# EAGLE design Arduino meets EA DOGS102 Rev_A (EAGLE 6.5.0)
Assembly variants: 3.3V monochrome, 3.3V RGB
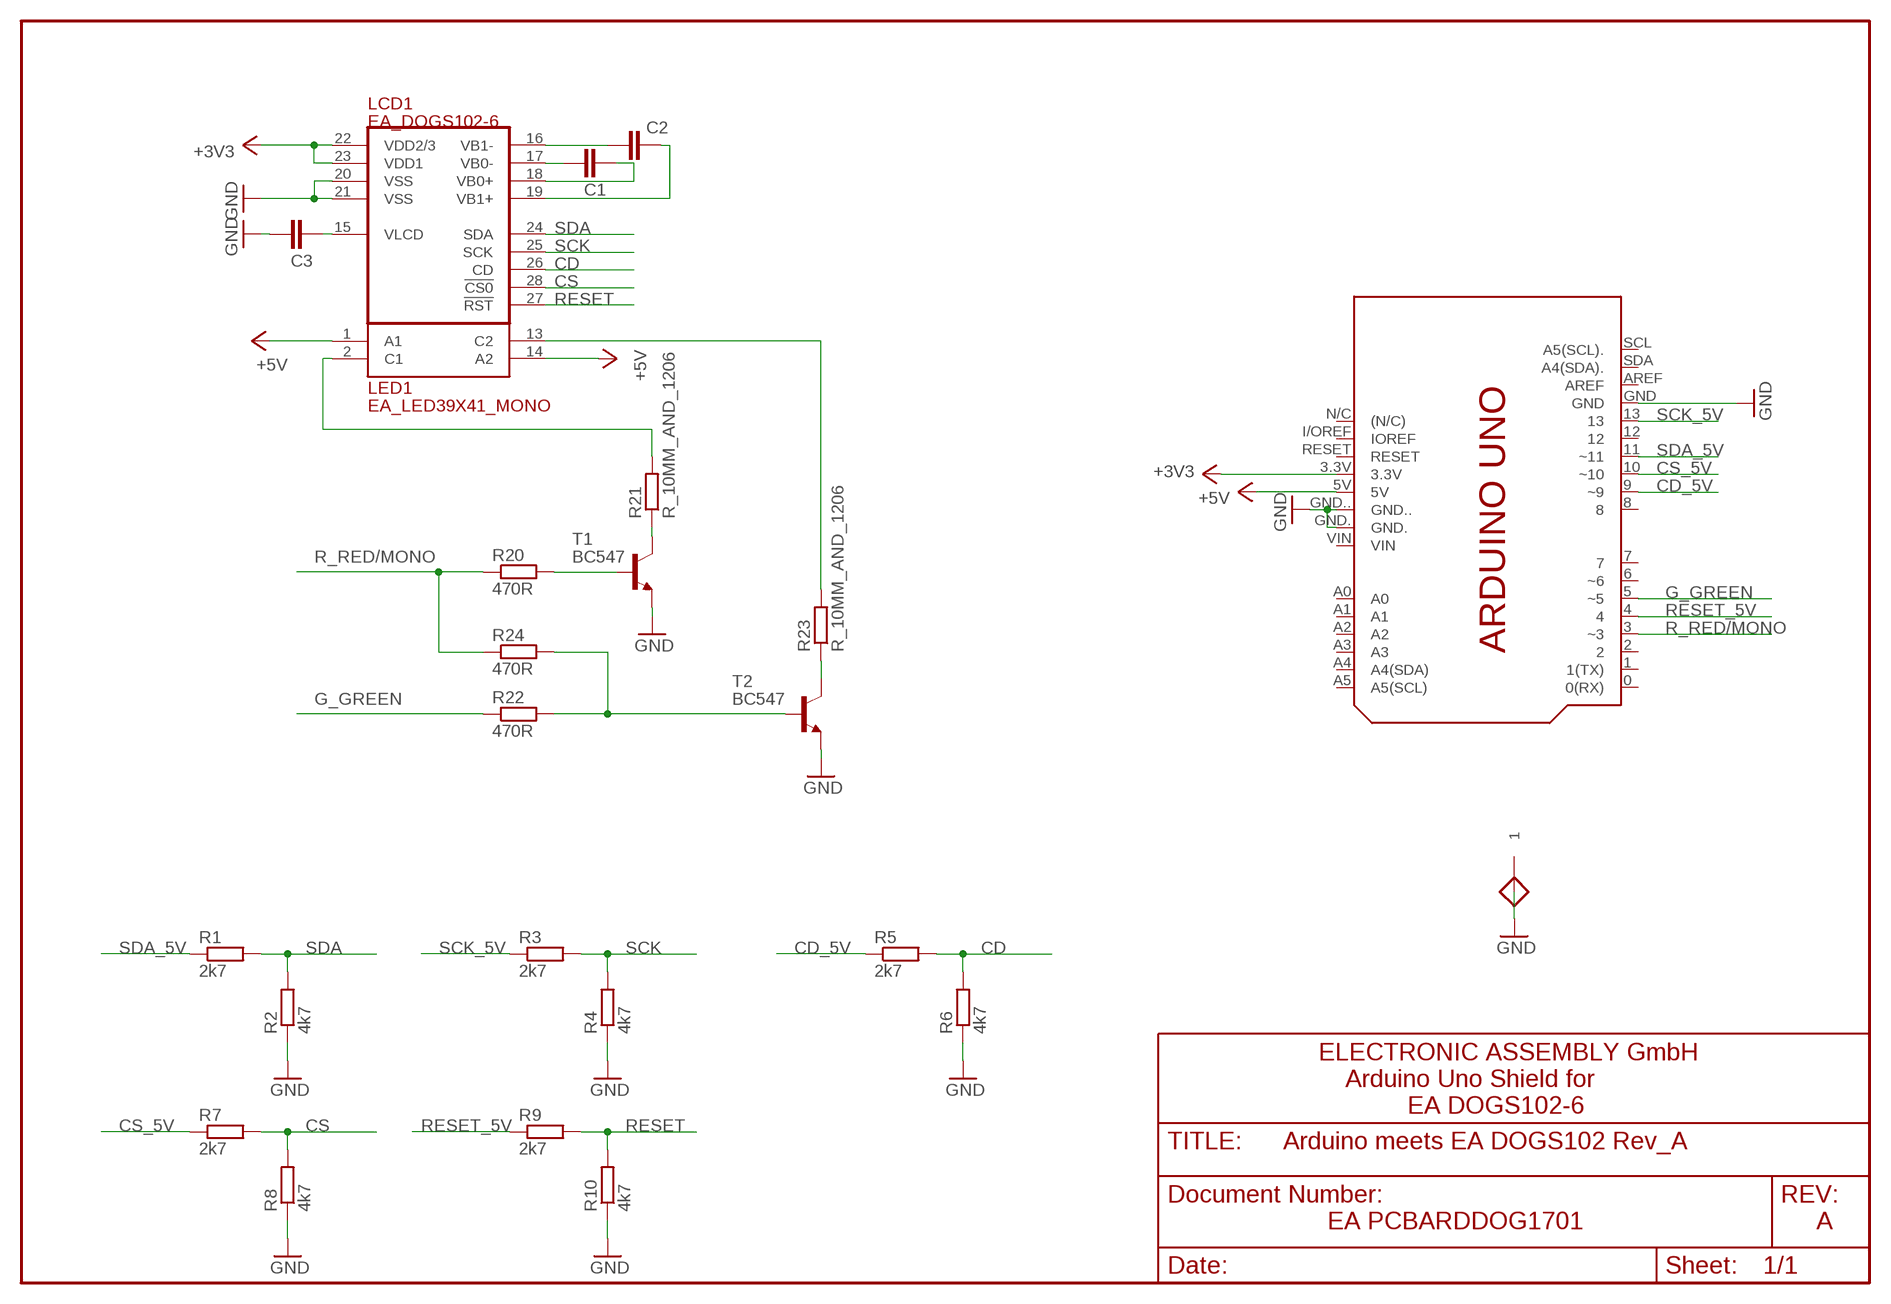
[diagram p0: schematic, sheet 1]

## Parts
C1  1uF  C_5MM_AND_1206  [C_5MM_AND_1206]
C2  1uF  C_5MM_AND_1206  [C_5MM_AND_1206]
C3  1uF  C_5MM_AND_1206  [C_5MM_AND_1206]
GND  PAD55/35  [PAD55/35]
LCD1  EA_DOGS102-6  [EA_DOGS102-6]
LED1  EA_LED39X41_MONO  [EA_LED39X41]
PCB1  ARDUINO_UNO_SHIELD  [ARDUINO_UNO_SHIELD]
R1  2k7  R_10MM_AND_1206  [R_10MM_AND_1206]
R2  4k7  R_10MM_AND_1206  [R_10MM_AND_1206]
R3  2k7  R_10MM_AND_1206  [R_10MM_AND_1206]
R4  4k7  R_10MM_AND_1206  [R_10MM_AND_1206]
R5  2k7  R_10MM_AND_1206  [R_10MM_AND_1206]
R6  4k7  R_10MM_AND_1206  [R_10MM_AND_1206]
R7  2k7  R_10MM_AND_1206  [R_10MM_AND_1206]
R8  4k7  R_10MM_AND_1206  [R_10MM_AND_1206]
R9  2k7  R_10MM_AND_1206  [R_10MM_AND_1206]
R10  4k7  R_10MM_AND_1206  [R_10MM_AND_1206]
R20  470R  R_10MM_AND_1206  [R_10MM_AND_1206]
R21  R_10MM_AND_1206  [R_10MM_AND_1206]
R22  470R  R_10MM_AND_1206  [R_10MM_AND_1206]  (not fitted in variant 3.3V monochrome)
R23  R_10MM_AND_1206  [R_10MM_AND_1206]
R24  470R  R_10MM_AND_1206  [R_10MM_AND_1206]  (not fitted in variant 3.3V RGB)
T1  BC547  [TO92]
T2  BC547  [TO92]

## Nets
+3V3: LCD1.22(VDD2/3) LCD1.23(VDD1) PCB1.3.3V
+5V: LED1.1(A1) LED1.14(A2) PCB1.5V
CD: LCD1.26(CD) R5.2 R6.2
CD_5V: PCB1.9(~9) R5.1
CS: LCD1.28(!CS0!) R7.2 R8.2
CS_5V: PCB1.10(~10) R7.1
G_GREEN: PCB1.5(~5) R22.1
GND: C3.2 GND.1 LCD1.20(VSS) LCD1.21(VSS) PCB1.GND PCB1.GND. PCB1.GND.. R2.1 R4.1 R6.1 R8.1 R10.1 T1.1(E) T2.1(E)
N$1: C1.2 LCD1.17(VB0-)
N$2: C2.2 LCD1.16(VB1-)
N$3: C1.1 LCD1.18(VB0+)
N$4: C2.1 LCD1.19(VB1+)
N$5: C3.1 LCD1.15(VLCD)
N$6: R21.1 T1.3(C)
N$7: LED1.2(C1) R21.2
N$12: R20.2 T1.2(B)
N$14: LED1.13(C2) R23.2
N$16: R23.1 T2.3(C)
N$17: R22.2 R24.2 T2.2(B)
R_RED/MONO: PCB1.3(~3) R20.1 R24.1
RESET: LCD1.27(!RST!) R9.2 R10.2
RESET_5V: PCB1.4 R9.1
SCK: LCD1.25(SCK) R3.2 R4.2
SCK_5V: PCB1.13 R3.1
SDA: LCD1.24(SDA) R1.2 R2.2
SDA_5V: PCB1.11(~11) R1.1
Unconnected: PCB1.0(0(RX)) PCB1.1(1(TX)) PCB1.2 PCB1.6(~6) PCB1.7 PCB1.8 PCB1.12 PCB1.A0 PCB1.A1 PCB1.A2 PCB1.A3 PCB1.A4(A4(SDA)) PCB1.A5(A5(SCL)) PCB1.AREF PCB1.I/OREF(IOREF) PCB1.N/C((N/C)) PCB1.RESET PCB1.SCL(A5(SCL).) PCB1.SDA(A4(SDA).) PCB1.VIN

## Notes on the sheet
- ELECTRONIC ASSEMBLY GmbH
- Arduino Uno Shield for
- EA DOGS102-6
- EA PCBARDDOG1701 | A

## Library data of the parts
C1-C3 = EA:C_5MM_AND_1206
GND = EA:PAD55/35
LCD1 = EA:EA_DOGS102-6
LED1 = EA:EA_LED39X41_MONO: Manufacturer: ELECTRONIC ASSEMBLY GmbH EA LED39x41-A EA LED39x41-W EA LED39x41-GR
PCB1 = E14_Arduino:ARDUINO_UNO_SHIELD
R1-R10 R20-R24 = EA:R_10MM_AND_1206
T1 T2 = transistor-npn:BC547: NPN TRANSISTOR

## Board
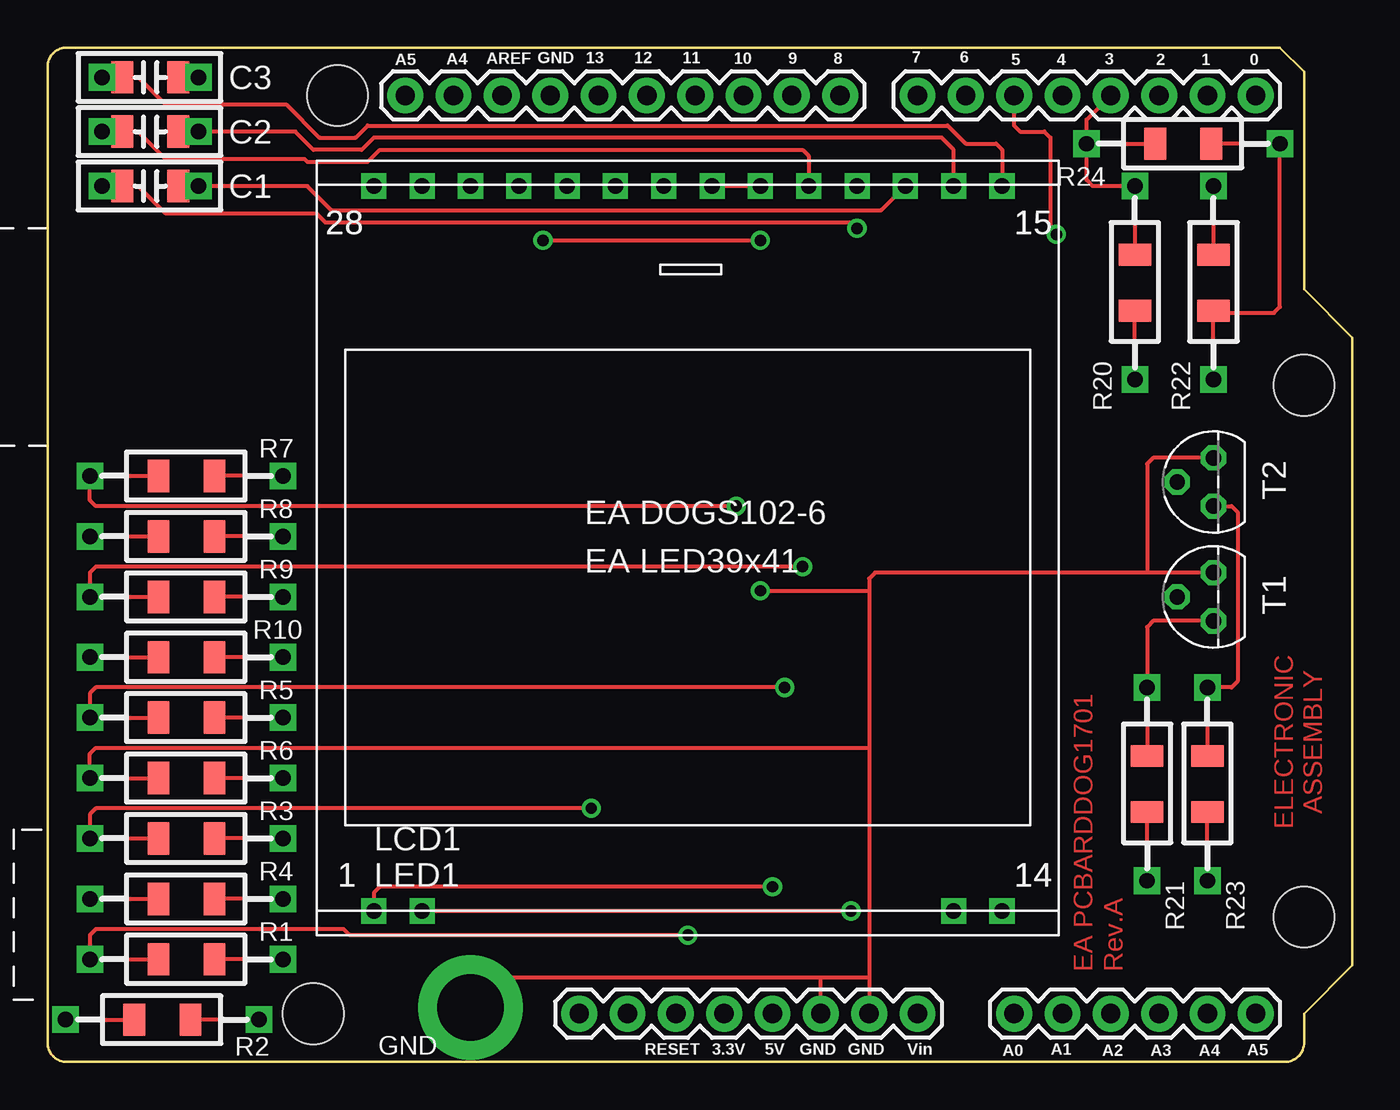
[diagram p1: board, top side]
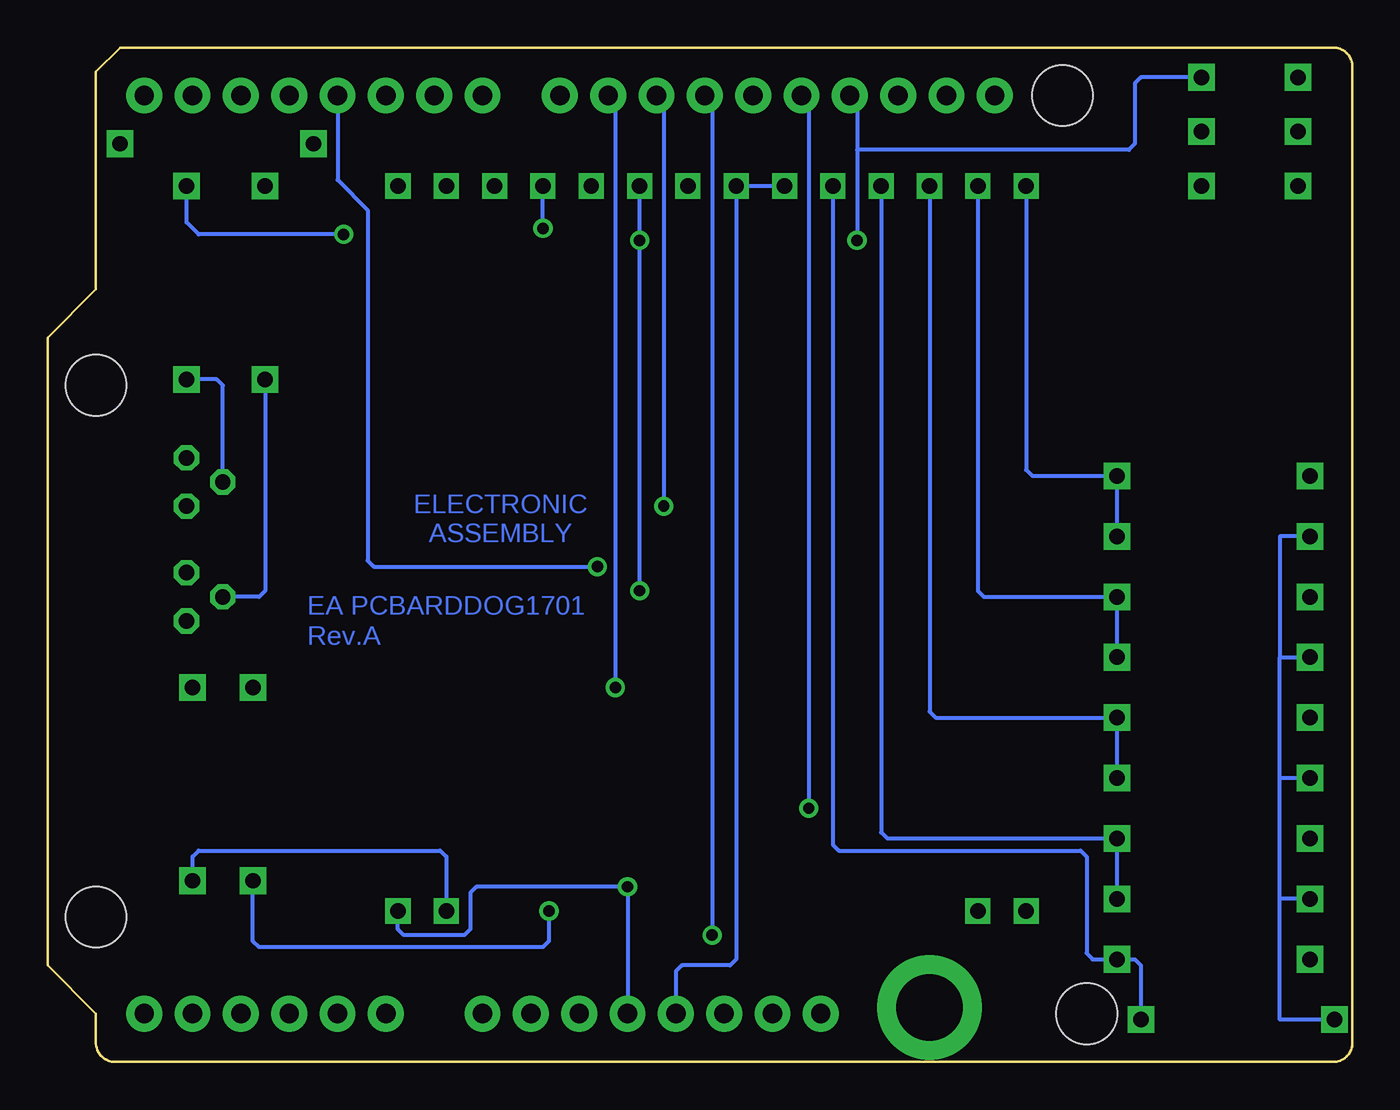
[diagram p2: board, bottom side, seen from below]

Size 68.58 x 53.31 mm. Coordinates in mm from the lower left corner, seen from the top.
Outline: 66.04,2.54 66.04,1.02 arc-90 65.02,0 1.02,0 arc-90 0,1.02 0,52.3 arc-90 1.02,53.31 64.77,53.31 66.04,52.05 66.04,40.62 68.58,38.08 68.58,5.08 66.04,2.54
Copper layers (1*16): Top 0.035mm / dielectric 1.5mm / Bottom 0.035mm
Design rules "default *": minimum track width 8mil, minimum drill 23mil, track to track 8mil, track to pad 8mil, pad to pad 8mil, via to via 8mil, smd to smd 8mil, copper to edge 40mil, drill to drill 8mil, minimum pad ring 10mil, minimum via ring 8mil, stop-mask expansion 4mil, vias tented up to drill 0mil, thermal gap 10mil

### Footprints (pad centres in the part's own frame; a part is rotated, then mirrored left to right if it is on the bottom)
C_5MM_AND_1206 = drill 0.813 pad 1.397 square: 1 0,0; 2 5.08,0 | smd 1.143 x 1.702: 3 4.013,0; 4 1.067,0
PAD55/35 = drill 3.5 pad 5.5: 1 0,0
EA_DOGS102-6 = drill 0.813 square: 1 0,0; 2 2.54,0; 13 30.48,0; 14 33.02,0; 15 33.02,38.1; 16 30.48,38.1; 17 27.94,38.1; 18 25.4,38.1; 19 22.86,38.1; 20 20.32,38.1; 21 17.78,38.1; 22 15.24,38.1; 23 12.7,38.1; 24 10.16,38.1; 25 7.62,38.1; 26 5.08,38.1; 27 2.54,38.1; 28 0,38.1
EA_LED39X41 = drill 0.813 square: 1 0,0; 2 2.54,0; 13 30.48,0; 14 33.02,0; 15 33.02,38.1; 16 30.48,38.1; 17 27.94,38.1; 18 25.4,38.1; 19 22.86,38.1; 20 20.32,38.1; 21 17.78,38.1; 22 15.24,38.1; 23 12.7,38.1; 24 10.16,38.1; 25 7.62,38.1; 26 5.08,38.1; 27 2.54,38.1; 28 0,38.1
ARDUINO_UNO_SHIELD = drill 1.016 pad 1.88: 0 63.5,50.8; 1 60.96,50.8; 2 58.42,50.8; 3 55.88,50.8; 3.3V 35.56,2.54; 4 53.34,50.8; 5 50.8,50.8; 5V 38.1,2.54; 6 48.26,50.8; 7 45.72,50.8; 8 41.656,50.8; 9 39.116,50.8; 10 36.576,50.8; 11 34.036,50.8; 12 31.496,50.8; 13 28.956,50.8; A0 50.8,2.54; A1 53.34,2.54; A2 55.88,2.54; A3 58.42,2.54; A4 60.96,2.54; A5 63.5,2.54; AREF 23.876,50.8; GND 26.416,50.8; GND. 43.18,2.54; GND.. 40.64,2.54; I/OREF 30.48,2.54; N/C 27.94,2.54; RESET 33.02,2.54; SCL 18.796,50.8; SDA 21.336,50.8; VIN 45.72,2.54 | hole 3.2: 66.04,7.62; 66.04,35.56; 15.24,50.8; 13.97,2.54
R_10MM_AND_1206 = drill 0.813 pad 1.397 square: 1 0,0; 2 10.16,0 | smd 1.143 x 1.702: 3 6.553,0; 4 3.607,0
TO92 = drill 0.813 octagon: 1 1.27,0; 2 0,1.905; 3 -1.27,0

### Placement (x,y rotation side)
C1  2.86,46.04 0 top
C2  2.86,48.9 0 top
C3  2.86,51.75 0 top
GND  22.23,2.86 0 top
LCD1  17.14,7.94 0 top
LED1  17.14,7.94 0 top
PCB1  0,0 0 top
R1  2.22,5.4 0 top
R2  0.95,2.22 0 top
R3  2.22,11.75 0 top
R4  2.22,8.57 0 top
R5  2.22,18.1 0 top
R6  2.22,14.92 0 top
R7  2.22,30.8 0 top
R8  2.22,27.62 0 top
R9  2.22,24.45 0 top
R10  2.22,21.27 0 top
R20  57.15,46.04 270 top
R21  57.78,19.68 270 top
R22  61.28,46.04 270 top
R23  60.96,19.68 270 top
R24  54.61,48.26 0 top
T1  61.28,24.45 90 top
T2  61.28,30.48 90 top

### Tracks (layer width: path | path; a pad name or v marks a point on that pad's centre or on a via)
+3V3
  Bottom 0.203: LCD1.23 LCD1.22 32.38,5.4 32.7,5.08 35.24,5.08 35.56,4.76 PCB1.3.3V
+5V  (via drill 0.6)
  Top 0.203: v38.1,9.21 17.46,9.21 17.14,8.89 LED1.1
  Bottom 0.203: PCB1.5V v38.1,9.21 46.04,9.21 46.35,8.89 46.35,6.99 46.67,6.67 49.85,6.67 50.16,6.99 LED1.14
CD
  Bottom 0.203: LCD1.26 22.23,18.41 21.91,18.1 R5.2 R6.2
CD_5V  (via drill 0.6)
  Top 0.203: v38.73,19.68 2.54,19.68 2.22,19.37 R5.1
  Bottom 0.203: PCB1.9 38.73,50.42 v38.73,19.68
CS
  Bottom 0.203: LCD1.28 17.14,31.11 16.83,30.8 R7.2 R8.2
CS_5V  (via drill 0.6)
  Top 0.203: v36.2,29.21 2.54,29.21 2.22,29.53 R7.1
  Bottom 0.203: PCB1.10 36.2,50.42 v36.2,29.21
G_GREEN  (via drill 0.6)
  Top 0.203: v53.02,43.5 52.7,43.81 52.7,48.58 52.39,48.9 51.12,48.9 50.8,49.21 PCB1.5
  Bottom 0.203: v53.02,43.5 60.64,43.5 61.28,44.13 R22.1
GND  (via drill 0.6)
  Top 0.203: GND.1 24.45,4.45 40.64,4.45 | PCB1.GND.. 40.64,4.45 | T1.1 57.78,25.72 | 57.78,25.72 43.5,25.72 43.18,25.4 43.18,24.77 | 43.18,24.77 43.18,16.51 | 43.18,16.51 43.18,4.45 | 43.18,4.45 PCB1.GND. | 40.64,4.45 43.18,4.45 | LCD1.20 LCD1.21 | R6.1 2.22,16.19 2.54,16.51 43.18,16.51 | v26.04,43.18 v37.47,43.18 | T2.1 58.1,31.75 57.78,31.43 57.78,25.72 | v37.47,24.77 43.18,24.77
  Bottom 0.203: R8.1 3.81,27.62 3.81,21.27 | 3.81,21.27 R10.1 | R6.1 3.81,14.92 | 3.81,14.92 3.81,21.27 | R4.1 3.81,8.57 | 3.81,8.57 3.81,14.92 | R2.1 3.81,2.22 3.81,8.57 | v37.47,24.77 v37.47,43.18 LCD1.20 | PCB1.GND 26.04,50.42 26.04,47.94 | 26.04,47.94 v26.04,43.18 | C3.2 11.11,51.75 11.43,51.44 11.43,48.26 11.75,47.94 26.04,47.94
N$1
  Top 0.203: LCD1.17 43.81,44.77 14.92,44.77 13.65,46.04 C1.2
N$2
  Top 0.203: LCD1.16 47.62,47.94 46.99,48.58 17.14,48.58 16.51,47.94 13.97,47.94 13.02,48.9 C2.2
N$3  (via drill 0.6)
  Top 0.203: v42.55,43.81 42.23,44.13 14.61,44.13 14.13,44.61 6.19,44.61 4.76,46.04 C1.1
  Bottom 0.203: v42.55,43.81 LCD1.18
N$4
  Top 0.203: C2.1 4.76,48.9 6.19,47.47 13.49,47.47 13.65,47.31 16.83,47.31 17.46,47.94 39.69,47.94 40.01,47.62 LCD1.19
N$5
  Top 0.203: C3.1 4.76,51.75 6.19,50.32 12.54,50.32 14.29,48.58 16.19,48.58 16.83,49.21 47.31,49.21 48.26,48.26 49.85,48.26 50.16,47.94 LCD1.15
N$6
  Top 0.203: T1.3 58.1,23.18 57.78,22.86 R21.1
N$7  (via drill 0.6)
  Top 0.203: LED1.2 v42.23,7.94
  Bottom 0.203: v42.23,7.94 42.23,6.35 42.55,6.03 57.47,6.03 57.78,6.35 R21.2
N$12
  Bottom 0.203: R20.2 57.15,24.77 57.47,24.45 T1.2
N$14
  Bottom 0.203: R23.2 60.96,10.79 60.64,11.11 47.94,11.11 47.62,10.79 LED1.13
N$16
  Top 0.203: T2.3 62.23,29.21 62.55,28.89 62.55,20 62.23,19.68 R23.1
N$17
  Top 0.203: 61.28,39.05 61.28,39.37 64.45,39.37 64.77,39.69 R24.2
  Bottom 0.203: T2.2 59.37,35.56 59.69,35.88 R22.2
R_RED/MONO
  Top 0.203: PCB1.3 54.61,49.53 R24.1 54.61,46.35 54.93,46.04 R20.1
RESET
  Bottom 0.203: LCD1.27 19.68,24.77 19.37,24.45 R9.2 R10.2
RESET_5V  (via drill 0.6)
  Top 0.203: v39.69,26.04 2.54,26.04 2.22,25.72 R9.1
  Bottom 0.203: PCB1.4 53.34,46.35 51.75,44.77 51.75,26.35 51.44,26.04 v39.69,26.04
SCK
  Bottom 0.203: LCD1.25 24.77,12.06 24.45,11.75 R3.2 R4.2
SCK_5V  (via drill 0.6)
  Top 0.203: v28.57,13.34 2.54,13.34 2.22,13.02 R3.1
  Bottom 0.203: PCB1.13 28.57,50.42 v28.57,13.34
SDA
  Bottom 0.203: LCD1.24 27.3,11.43 26.99,11.11 14.29,11.11 13.97,10.79 13.97,5.71 13.65,5.4 R1.2 11.43,5.4 11.11,5.08 R2.2
SDA_5V  (via drill 0.6)
  Top 0.203: v33.66,6.67 15.88,6.67 15.56,6.99 2.54,6.99 2.22,6.67 R1.1
  Bottom 0.203: PCB1.11 33.66,50.42 v33.66,6.67

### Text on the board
Top: ELECTRONIC / ASSEMBLY | EA PCBARDDOG1701 | Rev.A
Bottom: ELECTRONIC / ASSEMBLY | EA PCBARDDOG1701 | Rev.A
